|   stm32f427_437_429_439_tfbga216 IBIS Model
[IBIS ver]   4.2
[File name]  stm32f427_437_429_439_tfbga216.ibs
[File Rev]   1.3
[Date]   05-30-2014
[Source] Data Created at STMicroelectronics
[Notes]   File originated from ELDO simulations.
[Disclaimer]  This information is for modeling purpose only and is
   not guaranted. The information is subject to change without
   notice.
[Copyright] Copyright 2014 STMicroelectronics Inc.
[Component] stm32f427_437_429_439_tfbga216
[Manufacturer] STMicroelectronics
[Package]
| variable   typ   min   max
R_pkg   0.0   NA   NA
L_pkg   0.0H   NA   NA
C_pkg   0.0F   NA   NA
[Pin]   signal_name   model_name   R_pin   L_pin   C_pin
A3   PE2   io8p_arsudq_ft
A2   PE3   io8p_arsudq_ft
A1   PE4   io8p_arsudq_ft
B1   PE5   io8p_arsudq_ft
B2   PE6   io8p_arsudq_ft
G6   VSS   GND
F5   VDD   POWER
C1   VBAT   POWER
C2   PI8   io8p_arsudq_ft_v33
D1   PC13   io8p_arwsudq_ft_v33
E1   PC14   io8p_arwsudq_ft
F1   PC15   io8p_arsudq_ft
G5   VDD   POWER
E4   PI9   io8p_arsudq_ft
D5   PI10   io8p_arsudq_ft
F3   PI11   io8p_arsudq_ft
F2   VSS   GND
F4   VDD   POWER
D2   PF0   io8p_arsudq_i2cin_ft
E2   PF1   io8p_arsudq_i2cin_ft
G2   PF2   io8p_arsudq_ft
E3   PI12   io8p_arsudq_ft
G3   PI13   io8p_arsudq_ft
H3   PI14   io8p_arsudq_ft
H2   PF3   io8p_arwsudq_ft
J2   PF4   io8p_arwsudq_ft
K3   PF5   io8p_arwsudq_ft
H6   VSS   GND
H5   VDD   POWER
K2   PF6   io8p_arwsudq_ft
K1   PF7   io8p_arwsudq_ft
L3   PF8   io8p_arwsudq_ft
L2   PF9   io8p_arwsudq_ft
L1   PF10   io8p_arwsudq_ft
G1   PH0   io8p_arsudq_ft
H1   PH1   io8p_arsudq_ft
J1   NRST   ioreset_ft_v33
M2   PC0   io8p_ar3wsudq_ft
M3   PC1   io8p_ar3wsudq_ft
M4   PC2   io8p_ar3wsudq_ft
L4   PC3   io8p_ar3wsudq_ft
J5   VDD   POWER
J6   VSS   GND
M1   VSSA  GND
N1   VREFM   POWER
P1   VREFP   POWER
R1   VDDA   POWER
N3   PA0   io8p_ar3wsudq_ft_v33
N2   PA1   io8p_ar3wsudq_ft
P2   PA2   io8p_ar3wsudq_ft
K4   PH2   io8p_arsudq_ft
J4   PH3   io8p_arsudq_ft
H4   PH4   io8p_arsudq_i2cin_ft
J3   PH5   io8p_arsudq_i2cin_ft
R2   PA3   io8p_ar3wsudq_ft
K6   VSS   GND
L5   BYPASS_REG io8p_arsudq_ft_v33
K5   VDD   POWER
N4   PA4   io8p_ar3wsudq_ft
P4   PA5   io8p_ar3wsudq_ft
P3   PA6   io8p_ar3wsudq_ft
R3   PA7   io8p_ar3wsudq_ft
N5   PC4   io8p_ar3wsudq_ft
P5   PC5   io8p_ar3wsudq_ft
L7   VDD   POWER
L6   VSS   GND
R5   PB0   io8p_ar3wsudq_ft
R4   PB1   io8p_ar3wsudq_ft
M5   PB2   io8p_ar3wsudq_ft
G4   PI15   io8p_arsudq_ft
R6   PJ0   io8p_arsudq_ft
R7   PJ1   io8p_arsudq_ft
P7   PJ2   io8p_arsudq_ft
N8   PJ3   io8p_arsudq_ft
M9   PJ4   io8p_arsudq_ft
P8   PF11   io8p_arsudq_ft
M6   PF12   io8p_arsudq_ft
K7   VSS   GND
L8   VDD   POWER
N6   PF13   io8p_arsudq_ft
P6   PF14   io8p_arsudq_ft
M8   PF15   io8p_arsudq_ft
N7   PG0   io8p_arsudq_ft
M7   PG1   io8p_arsudq_ft
R8   PE7   io8p_arsudq_ft
N9   PE8   io8p_arsudq_ft
P9   PE9   io8p_arsudq_ft
K8   VSS   GND
L9   VDD   POWER
R9   PE10   io8p_arsudq_ft
P10   PE11   io8p_arsudq_ft
R10   PE12   io8p_arsudq_ft
R12   PE13   io8p_arsudq_ft
P11   PE14   io8p_arsudq_ft
R11   PE15   io8p_ar3wsudq_ft
P12   PB10   io8p_arsudq_i2cin_ft
R13   PB11   io8p_arsudq_i2cin_ft
L11   VCAP1   POWER
K9   VSS   GND
L10   VDD   POWER
M14   PJ5   io8p_arsudq_ft
P13   PH6   io8p_arsudq_ft
N13   PH7   io8p_arsudq_i2cin_ft
P14   PH8   io8p_arsudq_i2cin_ft
N14   PH9   io8p_arsudq_ft
p15   PH10   io8p_arsudq_ft
N15   PH11   io8p_arsudq_ft
M15   PH12   io8p_arsudq_ft
K10   VSS   GND
K11   VDD   POWER
L13   PB12   io8usb_id_otg_ft
K14   PB13   io8usb_vbus_otg_ft
R14   PB14   io8usb_lsfs_otg_ft
R15   PB15   io8usb_lsfs_otg_ft
L15   PD8   io8p_arsudq_ft
L14   PD9   io8p_arsudq_ft
K15   PD10   io8p_arsudq_ft
N10   PD11   io8p_arsudq_ft
M10   PD12   io8p_arsudq_ft
M11   PD13   io8p_arsudq_ft
J10   VSS   GND
J11   VDD   POWER
L12   PD14   io8p_arsudq_ft
K13   PD15   io8p_arsudq_ft
K12   PJ6   io8p_arsudq_ft
J12   PJ7   io8p_arsudq_ft
H12   PJ8   io8p_arsudq_ft
J13   PJ9   io8p_arsudq_ft
H13   PJ10   io8p_arsudq_ft
G12   PJ11   io8p_arsudq_ft
H11   VDD   POWER
H10   VSS   GND
G13   PK0   io8p_arsudq_ft
F12   PK1   io8p_arsudq_ft
F13   PK2   io8p_arsudq_ft
M13   PG2   io8p_arsudq_ft
M12   PG3   io8p_arsudq_ft
N12   PG4   io8p_arsudq_ft
N11   PG5   io8p_arsudq_ft
J15   PG6   io8p_arsudq_ft
J14   PG7   io8p_arsudq_ft
H14   PG8   io8p_arsudq_ft
G10   VSS   GND
G11   VDD   POWER
H15   PC6   io8p_arsudq_ft
G15   PC7   io8p_arsudq_ft
G14   PC8   io8p_arsudq_ft
F14   PC9   io8p_arsudq_i2cin_ft
F15   PA8   io8p_arsudq_i2cin_ft
E15   PA9   io8usb_vbus_otg_ft
D15   PA10   io8usb_id_otg_ft
C15   PA11   io8usb_lsfs_otg_ft
B15   PA12   io8usb_lsfs_otg_ft
A15   PA13   io8p_arsudq_ft
E11   VCAP2   POWER
F10   VSS   GND
F11   VDD   POWER
E12   PH13   io8p_arsudq_ft
E13   PH14   io8p_arsudq_ft
D13   PH15   io8p_arsudq_ft
E14   PI0   io8p_arsudq_ft
D14   PI1   io8p_arsudq_ft
C14   PI2   io8p_arsudq_ft
C13   PI3   io8p_arsudq_ft
F9   VSS   GND
E10   VDD   POWER
A14   PA14   io8p_arsudq_ft
A13   PA15   io8p_arsudq_ft
B14   PC10   io8p_arsudq_ft
B13   PC11   io8p_arsudq_ft
A12   PC12   io8p_arsudq_ft
B12   PD0   io8p_arsudq_ft
C12   PD1   io8p_arsudq_ft
D12   PD2   io8p_arsudq_ft
C11   PD3   io8p_arsudq_ft
D11   PD4   io8p_arsudq_ft
C10   PD5   io8p_arsudq_ft
F8   VSS   GND
E9   VDD   POWER
B11   PD6   io8p_arsudq_ft
A11   PD7   io8p_arsudq_ft
B10   PJ12   io8p_arsudq_ft
B9   PJ13   io8p_arsudq_ft
C9   PJ14   io8p_arsudq_ft
D10   PJ15   io8p_arsudq_ft
D9   PG9   io8p_arsudq_ft
C8   PG10   io8p_arsudq_ft
B8   PG11   io8p_arsudq_ft
C7   PG12   io8p_arsudq_ft
B3   PG13   io8p_arsudq_ft
A4   PG14   io8p_arsudq_ft
F7   VSS   GND
E8   VDD   POWER
D8   PK3   io8p_arsudq_ft
D7   PK4   io8p_arsudq_ft
C6   PK5   io8p_arsudq_ft
C5   PK6   io8p_arsudq_ft
C4   PK7   io8p_arsudq_ft
B7   PG15   io8p_arsudq_ft
A10   PB3   io8p_arsudq_ft
A9   PB4   io8p_arsudq_ft
A8   PB5   io8p_ar3wsudq_ft
B6   PB6   io8p_arsudq_i2cin_ft
B5   PB7   io8p_arsudq_i2cin_ft
E6   BOOT0   vpp_test_hv
A7   PB8   io8p_arsudq_i2cin_ft
B4   PB9   io8p_arsudq_i2cin_ft
A6   PE0   io8p_arsudq_ft
A5   PE1   io8p_arsudq_ft
F6   VSS   GND
E5   PDR_ON   io8p_arsudq_ft_v33
E7   VDD   POWER
C3   PI4   io8p_arsudq_ft
D3   PI5   io8p_arsudq_ft
D6   PI6   io8p_arsudq_ft
D4   PI7   io8p_arsudq_ft
[Diff Pin]   inv_pin   vdiff   tdelay_typ  tdelay_min  tdelay_max
R14   R15   200mV   NA   NA   NA
B15   C15   200mV   NA   NA   NA
[Model Selector] io8p_ar3wsudq_ft
io8p00_ar3wsudq_ft_pd_lv  "SPEED00 1P8V, PD=40kOhm"
io8p00_ar3wsudq_ft_pu_lv  "SPEED00 1P8V, PU=40kOhm"
io8p00_ar3wsudq_ft_lv   "SPEED00 1P8V"
io8p01_ar3wsudq_ft_pd_lv  "SPEED01 1P8V, PD=40kOhm"
io8p01_ar3wsudq_ft_pu_lv  "SPEED01 1P8V, PU=40kOhm"
io8p01_ar3wsudq_ft_lv  "SPEED01 1P8V"
io8p10_ar3wsudq_ft_pd_lv  "SPEED10 1P8V, PD=40kOhm"
io8p10_ar3wsudq_ft_pu_lv  "SPEED10 1P8V, PU=40kOhm"
io8p10_ar3wsudq_ft_lv  "SPEED10 1P8V"
io8p11_ar3wsudq_ft_pd_lv  "SPEED11 1P8V, PD=40kOhm"
io8p11_ar3wsudq_ft_pu_lv  "SPEED11 1P8V, PU=40kOhm"
io8p11_ar3wsudq_ft_lv  "SPEED11 1P8V"
io8p00_ar3wsudq_ft_pd  "SPEED00, PD=40kOhm"
io8p00_ar3wsudq_ft_pu  "SPEED00, PU=40kOhm"
io8p00_ar3wsudq_ft  "SPEED00"
io8p01_ar3wsudq_ft_pd  "SPEED01, PD=40kOhm"
io8p01_ar3wsudq_ft_pu  "SPEED01, PU=40kOhm"
io8p01_ar3wsudq_ft  "SPEED01"
io8p10_ar3wsudq_ft_pd  "SPEED10, PD=40kOhm"
io8p10_ar3wsudq_ft_pu  "SPEED10, PU=40kOhm"
io8p10_ar3wsudq_ft  "SPEED10"
io8p11_ar3wsudq_ft_pd  "SPEED11, PD=40kOhm"
io8p11_ar3wsudq_ft_pu  "SPEED11, PU=40kOhm"
io8p11_ar3wsudq_ft  "SPEED11"
[Model Selector] io8p_ar3wsudq_ft_v33
io8p00_ar3wsudq_ft_v33_pd_lv  "SPEED00 1P8V, PD=40kOhm"
io8p00_ar3wsudq_ft_v33_pu_lv  "SPEED00 1P8V, PU=40kOhm"
io8p00_ar3wsudq_ft_v33_lv  "SPEED00 1P8V"
io8p01_ar3wsudq_ft_v33_pd_lv  "SPEED01 1P8V, PD=40kOhm"
io8p01_ar3wsudq_ft_v33_pu_lv  "SPEED01 1P8V, PU=40kOhm"
io8p01_ar3wsudq_ft_v33_lv  "SPEED01 1P8V"
io8p10_ar3wsudq_ft_v33_pd_lv  "SPEED10 1P8V, PD=40kOhm"
io8p10_ar3wsudq_ft_v33_pu_lv  "SPEED10 1P8V, PU=40kOhm"
io8p10_ar3wsudq_ft_v33_lv  "SPEED10 1P8V"
io8p11_ar3wsudq_ft_v33_pd_lv  "SPEED11 1P8V, PD=40kOhm"
io8p11_ar3wsudq_ft_v33_pu_lv  "SPEED11 1P8V, PU=40kOhm"
io8p11_ar3wsudq_ft_v33_lv  "SPEED11 1P8V"
io8p00_ar3wsudq_ft_v33_pd  "SPEED00, PD=40kOhm"
io8p00_ar3wsudq_ft_v33_pu  "SPEED00, PU=40kOhm"
io8p00_ar3wsudq_ft_v33  "SPEED00"
io8p01_ar3wsudq_ft_v33_pd  "SPEED01, PD=40kOhm"
io8p01_ar3wsudq_ft_v33_pu  "SPEED01, PU=40kOhm"
io8p01_ar3wsudq_ft_v33  "SPEED01"
io8p10_ar3wsudq_ft_v33_pd  "SPEED10, PD=40kOhm"
io8p10_ar3wsudq_ft_v33_pu  "SPEED10, PU=40kOhm"
io8p10_ar3wsudq_ft_v33  "SPEED10"
io8p11_ar3wsudq_ft_v33_pd  "SPEED11, PD=40kOhm"
io8p11_ar3wsudq_ft_v33_pu  "SPEED11, PU=40kOhm"
io8p11_ar3wsudq_ft_v33  "SPEED11"
[Model Selector] io8p_arsudq_ft
io8p00_arsudq_ft_pd_lv  "SPEED00 1P8V, PD=40kOhm"
io8p00_arsudq_ft_pu_lv  "SPEED00 1P8V, PU=40kOhm"
io8p00_arsudq_ft_lv  "SPEED00 1P8V"
io8p01_arsudq_ft_pd_lv  "SPEED01 1P8V, PD=40kOhm"
io8p01_arsudq_ft_pu_lv  "SPEED01 1P8V, PU=40kOhm"
io8p01_arsudq_ft_lv  "SPEED01 1P8V"
io8p10_arsudq_ft_pd_lv  "SPEED10 1P8V, PD=40kOhm"
io8p10_arsudq_ft_pu_lv  "SPEED10 1P8V, PU=40kOhm"
io8p10_arsudq_ft_lv  "SPEED10 1P8V"
io8p11_arsudq_ft_pd_lv  "SPEED11 1P8V, PD=40kOhm"
io8p11_arsudq_ft_pu_lv  "SPEED11 1P8V, PU=40kOhm"
io8p11_arsudq_ft_lv  "SPEED11 1P8V"
io8p00_arsudq_ft_pd  "SPEED00, PD=40kOhm"
io8p00_arsudq_ft_pu  "SPEED00, PU=40kOhm"
io8p00_arsudq_ft  "SPEED00"
io8p01_arsudq_ft_pd  "SPEED01, PD=40kOhm"
io8p01_arsudq_ft_pu  "SPEED01, PU=40kOhm"
io8p01_arsudq_ft  "SPEED01"
io8p10_arsudq_ft_pd  "SPEED10, PD=40kOhm"
io8p10_arsudq_ft_pu  "SPEED10, PU=40kOhm"
io8p10_arsudq_ft  "SPEED10"
io8p11_arsudq_ft_pd  "SPEED11, PD=40kOhm"
io8p11_arsudq_ft_pu  "SPEED11, PU=40kOhm"
io8p11_arsudq_ft  "SPEED11"
[Model Selector] io8p_arsudq_ft_v33
io8p00_arsudq_ft_v33_pd_lv  "SPEED00 1P8V, PD=40kOhm"
io8p00_arsudq_ft_v33_pu_lv  "SPEED00 1P8V, PU=40kOhm"
io8p00_arsudq_ft_v33_lv  "SPEED00 1P8V"
io8p01_arsudq_ft_v33_pd_lv  "SPEED01 1P8V, PD=40kOhm"
io8p01_arsudq_ft_v33_pu_lv  "SPEED01 1P8V, PU=40kOhm"
io8p01_arsudq_ft_v33_lv  "SPEED01 1P8V"
io8p10_arsudq_ft_v33_pd_lv  "SPEED10 1P8V, PD=40kOhm"
io8p10_arsudq_ft_v33_pu_lv  "SPEED10 1P8V, PU=40kOhm"
io8p10_arsudq_ft_v33_lv  "SPEED10 1P8V"
io8p11_arsudq_ft_v33_pd_lv  "SPEED11 1P8V, PD=40kOhm"
io8p11_arsudq_ft_v33_pu_lv  "SPEED11 1P8V, PU=40kOhm"
io8p11_arsudq_ft_v33_lv  "SPEED11 1P8V"
io8p00_arsudq_ft_v33_pd  "SPEED00, PD=40kOhm"
io8p00_arsudq_ft_v33_pu  "SPEED00, PU=40kOhm"
io8p00_arsudq_ft_v33  "SPEED00"
io8p01_arsudq_ft_v33_pd  "SPEED01, PD=40kOhm"
io8p01_arsudq_ft_v33_pu  "SPEED01, PU=40kOhm"
io8p01_arsudq_ft_v33  "SPEED01"
io8p10_arsudq_ft_v33_pd  "SPEED10, PD=40kOhm"
io8p10_arsudq_ft_v33_pu  "SPEED10, PU=40kOhm"
io8p10_arsudq_ft_v33  "SPEED10"
io8p11_arsudq_ft_v33_pd  "SPEED11, PD=40kOhm"
io8p11_arsudq_ft_v33_pu  "SPEED11, PU=40kOhm"
io8p11_arsudq_ft_v33  "SPEED11"
[Model Selector] io8p_arsudq_i2cin_ft
io8p00_arsudq_i2cin_ft_pd_lv  "SPEED00 1P8V, PD=40kOhm"
io8p00_arsudq_i2cin_ft_pu_lv  "SPEED00 1P8V, PU=40kOhm"
io8p00_arsudq_i2cin_ft_lv  "SPEED00 1P8V"
io8p01_arsudq_i2cin_ft_pd_lv  "SPEED01 1P8V, PD=40kOhm"
io8p01_arsudq_i2cin_ft_pu_lv  "SPEED01 1P8V, PU=40kOhm"
io8p01_arsudq_i2cin_ft_lv  "SPEED01 1P8V"
io8p10_arsudq_i2cin_ft_pd_lv  "SPEED10 1P8V, PD=40kOhm"
io8p10_arsudq_i2cin_ft_pu_lv  "SPEED10 1P8V, PU=40kOhm"
io8p10_arsudq_i2cin_ft_lv  "SPEED10 1P8V"
io8p11_arsudq_i2cin_ft_pd_lv  "SPEED11 1P8V, PD=40kOhm"
io8p11_arsudq_i2cin_ft_pu_lv  "SPEED11 1P8V, PU=40kOhm"
io8p11_arsudq_i2cin_ft_lv  "SPEED11 1P8V"
io8p00_arsudq_i2cin_ft_pd  "SPEED00, PD=40kOhm"
io8p00_arsudq_i2cin_ft_pu  "SPEED00, PU=40kOhm"
io8p00_arsudq_i2cin_ft  "SPEED00"
io8p01_arsudq_i2cin_ft_pd  "SPEED01, PD=40kOhm"
io8p01_arsudq_i2cin_ft_pu  "SPEED01, PU=40kOhm"
io8p01_arsudq_i2cin_ft  "SPEED01"
io8p10_arsudq_i2cin_ft_pd  "SPEED10, PD=40kOhm"
io8p10_arsudq_i2cin_ft_pu  "SPEED10, PU=40kOhm"
io8p10_arsudq_i2cin_ft  "SPEED10"
io8p11_arsudq_i2cin_ft_pd  "SPEED11, PD=40kOhm"
io8p11_arsudq_i2cin_ft_pu  "SPEED11, PU=40kOhm"
io8p11_arsudq_i2cin_ft  "SPEED11"
[Model Selector] io8p_arwsudq_ft
io8p00_arwsudq_ft_pd_lv  "SPEED00 1P8V, PD=40kOhm"
io8p00_arwsudq_ft_pu_lv  "SPEED00 1P8V, PU=40kOhm"
io8p00_arwsudq_ft_lv  "SPEED00 1P8V"
io8p01_arwsudq_ft_pd_lv  "SPEED01 1P8V, PD=40kOhm"
io8p01_arwsudq_ft_pu_lv  "SPEED01 1P8V, PU=40kOhm"
io8p01_arwsudq_ft_lv  "SPEED01 1P8V"
io8p10_arwsudq_ft_pd_lv  "SPEED10 1P8V, PD=40kOhm"
io8p10_arwsudq_ft_pu_lv  "SPEED10 1P8V, PU=40kOhm"
io8p10_arwsudq_ft_lv  "SPEED10 1P8V"
io8p11_arwsudq_ft_pd_lv  "SPEED11 1P8V, PD=40kOhm"
io8p11_arwsudq_ft_pu_lv  "SPEED11 1P8V, PU=40kOhm"
io8p11_arwsudq_ft_lv  "SPEED11 1P8V"
io8p00_arwsudq_ft_pd  "SPEED00, PD=40kOhm"
io8p00_arwsudq_ft_pu  "SPEED00, PU=40kOhm"
io8p00_arwsudq_ft  "SPEED00"
io8p01_arwsudq_ft_pd  "SPEED01, PD=40kOhm"
io8p01_arwsudq_ft_pu  "SPEED01, PU=40kOhm"
io8p01_arwsudq_ft  "SPEED01"
io8p10_arwsudq_ft_pd  "SPEED10, PD=40kOhm"
io8p10_arwsudq_ft_pu  "SPEED10, PU=40kOhm"
io8p10_arwsudq_ft  "SPEED10"
io8p11_arwsudq_ft_pd  "SPEED11, PD=40kOhm"
io8p11_arwsudq_ft_pu  "SPEED11, PU=40kOhm"
io8p11_arwsudq_ft  "SPEED11"
[Model Selector] io8p_arwsudq_ft_v33
io8p00_arwsudq_ft_v33_pd_lv  "SPEED00 1P8V, PD=40kOhm"
io8p00_arwsudq_ft_v33_pu_lv  "SPEED00 1P8V, PU=40kOhm"
io8p00_arwsudq_ft_v33_lv  "SPEED00 1P8V"
io8p01_arwsudq_ft_v33_pd_lv  "SPEED01 1P8V, PD=40kOhm"
io8p01_arwsudq_ft_v33_pu_lv  "SPEED01 1P8V, PU=40kOhm"
io8p01_arwsudq_ft_v33_lv  "SPEED01 1P8V"
io8p10_arwsudq_ft_v33_pd_lv  "SPEED10 1P8V, PD=40kOhm"
io8p10_arwsudq_ft_v33_pu_lv  "SPEED10 1P8V, PU=40kOhm"
io8p10_arwsudq_ft_v33_lv  "SPEED10 1P8V"
io8p11_arwsudq_ft_v33_pd_lv  "SPEED11 1P8V, PD=40kOhm"
io8p11_arwsudq_ft_v33_pu_lv  "SPEED11 1P8V, PU=40kOhm"
io8p11_arwsudq_ft_v33_lv  "SPEED11 1P8V"
io8p00_arwsudq_ft_v33_pd  "SPEED00, PD=40kOhm"
io8p00_arwsudq_ft_v33_pu  "SPEED00, PU=40kOhm"
io8p00_arwsudq_ft_v33  "SPEED00"
io8p01_arwsudq_ft_v33_pd  "SPEED01, PD=40kOhm"
io8p01_arwsudq_ft_v33_pu  "SPEED01, PU=40kOhm"
io8p01_arwsudq_ft_v33  "SPEED01"
io8p10_arwsudq_ft_v33_pd  "SPEED10, PD=40kOhm"
io8p10_arwsudq_ft_v33_pu  "SPEED10, PU=40kOhm"
io8p10_arwsudq_ft_v33  "SPEED10"
io8p11_arwsudq_ft_v33_pd  "SPEED11, PD=40kOhm"
io8p11_arwsudq_ft_v33_pu  "SPEED11, PU=40kOhm"
io8p11_arwsudq_ft_v33  "SPEED11"
[Model Selector] io8usb_id_otg_ft
io8p00_id_otg_ft_pd_lv  "SPEED00 1P8V, PD=14kOhm"
io8p00_id_otg_ft_pu_lv  "SPEED00 1P8V, PU=14kOhm"
io8p00_id_otg_ft_lv  "SPEED00 1P8V"
io8p01_id_otg_ft_pd_lv  "SPEED01 1P8V, PD=14kOhm"
io8p01_id_otg_ft_pu_lv  "SPEED01 1P8V, PU=14kOhm"
io8p01_id_otg_ft_lv  "SPEED01 1P8V"
io8p10_id_otg_ft_pd_lv  "SPEED10 1P8V, PD=14kOhm"
io8p10_id_otg_ft_pu_lv  "SPEED10 1P8V, PU=14kOhm"
io8p10_id_otg_ft_lv  "SPEED10 1P8V"
io8p11_id_otg_ft_pd_lv  "SPEED11 1P8V, PD=14kOhm"
io8p11_id_otg_ft_pu_lv  "SPEED11 1P8V, PU=14kOhm"
io8p11_id_otg_ft_lv  "SPEED11 1P8V"
io8p00_id_otg_ft_pd  "SPEED00, PD=14kOhm"
io8p00_id_otg_ft_pu  "SPEED00, PU=14kOhm"
io8p00_id_otg_ft  "SPEED00"
io8p01_id_otg_ft_pd  "SPEED01, PD=14kOhm"
io8p01_id_otg_ft_pu  "SPEED01, PU=14kOhm"
io8p01_id_otg_ft  "SPEED01"
io8p10_id_otg_ft_pd  "SPEED10, PD=14kOhm"
io8p10_id_otg_ft_pu  "SPEED10, PU=14kOhm"
io8p10_id_otg_ft  "SPEED10"
io8p11_id_otg_ft_pd  "SPEED11, PD=14kOhm"
io8p11_id_otg_ft_pu  "SPEED11, PU=14kOhm"
io8p11_id_otg_ft  "SPEED11"
[Model Selector] io8usb_lsfs_otg_ft
io8usb_ls_otg_ft_dpdn_pd  "LS USB DP/DN IO + PD=20kOhm"
io8usb_ls_otg_ft_dpdn_pupu2  "LS USB DP/DN IO + PU/PU2=2.2kOhm"
io8usb_ls_otg_ft_dpdn_pu2  "LS USB DP/DN IO + PU2=1.2kOhm"
io8usb_ls_otg_ft_dpdn_pu  "LS USB DP/DN IO + PU=1.2kOhm"
io8usb_ls_otg_ft_dpdn  "LS USB DP/DN IO"
io8usb_fs_otg_ft_dpdn_pd  "HS USB DP/DN IO + PD=20kOhm"
io8usb_fs_otg_ft_dpdn_pupu2  "HS USB DP/DN IO + PU/PU2=2.2kOhm"
io8usb_fs_otg_ft_dpdn_pu2  "HS USB DP/DN IO + PU2=1.2kOhm"
io8usb_fs_otg_ft_dpdn_pu  "HS USB DP/DN IO + PU=1.2kOhm"
io8usb_fs_otg_ft_dpdn  "HS USB DP/DN IO"
io8p00_lsfs_otg_ft_pd_lv  "SPEED00 1P8V, PD=40kOhm"
io8p00_lsfs_otg_ft_pu_lv  "SPEED00 1P8V, PU=40kOhm"
io8p00_lsfs_otg_ft_lv  "SPEED00 1P8V"
io8p01_lsfs_otg_ft_pd_lv  "SPEED01 1P8V, PD=40kOhm"
io8p01_lsfs_otg_ft_pu_lv  "SPEED01 1P8V, PU=40kOhm"
io8p01_lsfs_otg_ft_lv  "SPEED01 1P8V"
io8p10_lsfs_otg_ft_pd_lv  "SPEED10 1P8V, PD=40kOhm"
io8p10_lsfs_otg_ft_pu_lv  "SPEED10 1P8V, PU=40kOhm"
io8p10_lsfs_otg_ft_lv  "SPEED10 1P8V"
io8p11_lsfs_otg_ft_pd_lv  "SPEED11 1P8V, PD=40kOhm"
io8p11_lsfs_otg_ft_pu_lv  "SPEED11 1P8V, PU=40kOhm"
io8p11_lsfs_otg_ft_lv  "SPEED11 1P8V"
io8p00_lsfs_otg_ft_pd  "SPEED00, PD=40kOhm"
io8p00_lsfs_otg_ft_pu  "SPEED00, PU=40kOhm"
io8p00_lsfs_otg_ft  "SPEED00"
io8p01_lsfs_otg_ft_pd  "SPEED01, PD=40kOhm"
io8p01_lsfs_otg_ft_pu  "SPEED01, PU=40kOhm"
io8p01_lsfs_otg_ft  "SPEED01"
io8p10_lsfs_otg_ft_pd  "SPEED10, PD=40kOhm"
io8p10_lsfs_otg_ft_pu  "SPEED10, PU=40kOhm"
io8p10_lsfs_otg_ft  "SPEED10"
io8p11_lsfs_otg_ft_pd  "SPEED11, PD=40kOhm"
io8p11_lsfs_otg_ft_pu  "SPEED11, PU=40kOhm"
io8p11_lsfs_otg_ft  "SPEED11"
[Model Selector] io8usb_vbus_otg_ft
io8psenb_vbus_otg_ft  "VBUS PULSE, SENSE VB"
io8psenab_vbus_otg_ft  "VBUS PULSE, SENSE VA and VB"
io8psena_vbus_otg_ft  "VBUS PULSE, SENSE VA"
io8psen_vbus_otg_ft  "VBUS PULSE"
io8p00_vbus_otg_ft_pd_lv  "SPEED00 1P8V, PD=40kOhm"
io8p00_vbus_otg_ft_pu_lv  "SPEED00 1P8V, PU=40kOhm"
io8p00_vbus_otg_ft_lv  "SPEED00 1P8V"
io8p01_vbus_otg_ft_pd_lv  "SPEED01 1P8V, PD=40kOhm"
io8p01_vbus_otg_ft_pu_lv  "SPEED01 1P8V, PU=40kOhm"
io8p01_vbus_otg_ft_lv  "SPEED01 1P8V"
io8p10_vbus_otg_ft_pd_lv  "SPEED10 1P8V, PD=40kOhm"
io8p10_vbus_otg_ft_pu_lv  "SPEED10 1P8V, PU=40kOhm"
io8p10_vbus_otg_ft_lv  "SPEED10 1P8V"
io8p11_vbus_otg_ft_pd_lv  "SPEED11 1P8V, PD=40kOhm"
io8p11_vbus_otg_ft_pu_lv  "SPEED11 1P8V, PU=40kOhm"
io8p11_vbus_otg_ft_lv  "SPEED11 1P8V"
io8p00_vbus_otg_ft_pd  "SPEED00, PD=40kOhm"
io8p00_vbus_otg_ft_pu  "SPEED00, PU=40kOhm"
io8p00_vbus_otg_ft  "SPEED00"
io8p01_vbus_otg_ft_pd  "SPEED01, PD=40kOhm"
io8p01_vbus_otg_ft_pu  "SPEED01, PU=40kOhm"
io8p01_vbus_otg_ft  "SPEED01"
io8p10_vbus_otg_ft_pd  "SPEED10, PD=40kOhm"
io8p10_vbus_otg_ft_pu  "SPEED10, PU=40kOhm"
io8p10_vbus_otg_ft  "SPEED10"
io8p11_vbus_otg_ft_pd  "SPEED11, PD=40kOhm"
io8p11_vbus_otg_ft_pu  "SPEED11, PU=40kOhm"
io8p11_vbus_otg_ft  "SPEED11"
[Model Selector] ioreset_ft_v33
ioreset_ft_v33_pu_lv  "ioreset 1P8V + PU=40kOhm"
ioreset_ft_v33_nopu_lv  "ioreset 1P8V"
ioreset_ft_v33_pu  "ioreset + PU=40kOhm"
ioreset_ft_v33_nopu  "ioreset"
[Model Selector] vpp_test_hv
vpp_test_hv_2p4  "Input Buffer 1P8V"
vpp_test_hv_3p3  "Input Buffer"
| Models and submodels in the file (260): io8p00_ar3wsudq_ft_pd_lv (I/O), io8p00_ar3wsudq_ft_pu_lv (I/O), io8p00_ar3wsudq_ft_lv (I/O), io8p01_ar3wsudq_ft_pd_lv (I/O), io8p01_ar3wsudq_ft_pu_lv (I/O), io8p01_ar3wsudq_ft_lv (I/O), io8p10_ar3wsudq_ft_pd_lv (I/O), io8p10_ar3wsudq_ft_pu_lv (I/O), io8p10_ar3wsudq_ft_lv (I/O), io8p11_ar3wsudq_ft_pd_lv (I/O), io8p11_ar3wsudq_ft_pu_lv (I/O), io8p11_ar3wsudq_ft_lv (I/O), io8p00_ar3wsudq_ft_pd (I/O), io8p00_ar3wsudq_ft_pu (I/O), io8p00_ar3wsudq_ft (I/O), io8p01_ar3wsudq_ft_pd (I/O), io8p01_ar3wsudq_ft_pu (I/O), io8p01_ar3wsudq_ft (I/O), io8p10_ar3wsudq_ft_pd (I/O), io8p10_ar3wsudq_ft_pu (I/O), io8p10_ar3wsudq_ft (I/O), io8p11_ar3wsudq_ft_pd (I/O), io8p11_ar3wsudq_ft_pu (I/O), io8p11_ar3wsudq_ft (I/O), io8p00_ar3wsudq_ft_v33_pd_lv (I/O), io8p00_ar3wsudq_ft_v33_pu_lv (I/O), io8p00_ar3wsudq_ft_v33_lv (I/O), io8p01_ar3wsudq_ft_v33_pd_lv (I/O), io8p01_ar3wsudq_ft_v33_pu_lv (I/O), io8p01_ar3wsudq_ft_v33_lv (I/O), io8p10_ar3wsudq_ft_v33_pd_lv (I/O), io8p10_ar3wsudq_ft_v33_pu_lv (I/O), io8p10_ar3wsudq_ft_v33_lv (I/O), io8p11_ar3wsudq_ft_v33_pd_lv (I/O), io8p11_ar3wsudq_ft_v33_pu_lv (I/O), io8p11_ar3wsudq_ft_v33_lv (I/O), io8p00_ar3wsudq_ft_v33_pd (I/O), io8p00_ar3wsudq_ft_v33_pu (I/O), io8p00_ar3wsudq_ft_v33 (I/O), io8p01_ar3wsudq_ft_v33_pd (I/O), io8p01_ar3wsudq_ft_v33_pu (I/O), io8p01_ar3wsudq_ft_v33 (I/O), io8p10_ar3wsudq_ft_v33_pd (I/O), io8p10_ar3wsudq_ft_v33_pu (I/O), io8p10_ar3wsudq_ft_v33 (I/O), io8p11_ar3wsudq_ft_v33_pd (I/O), io8p11_ar3wsudq_ft_v33_pu (I/O), io8p11_ar3wsudq_ft_v33 (I/O), io8p00_arsudq_ft_pd_lv (I/O), io8p00_arsudq_ft_pu_lv (I/O), io8p00_arsudq_ft_lv (I/O), io8p01_arsudq_ft_pd_lv (I/O), io8p01_arsudq_ft_pu_lv (I/O), io8p01_arsudq_ft_lv (I/O), io8p10_arsudq_ft_pd_lv (I/O), io8p10_arsudq_ft_pu_lv (I/O), io8p10_arsudq_ft_lv (I/O), io8p11_arsudq_ft_pd_lv (I/O), io8p11_arsudq_ft_pu_lv (I/O), io8p11_arsudq_ft_lv (I/O), io8p00_arsudq_ft_pd (I/O), io8p00_arsudq_ft_pu (I/O), io8p00_arsudq_ft (I/O), io8p01_arsudq_ft_pd (I/O), io8p01_arsudq_ft_pu (I/O), io8p01_arsudq_ft (I/O), io8p10_arsudq_ft_pd (I/O), io8p10_arsudq_ft_pu (I/O), io8p10_arsudq_ft (I/O), io8p11_arsudq_ft_pd (I/O), io8p11_arsudq_ft_pu (I/O), io8p11_arsudq_ft (I/O), io8p00_arsudq_ft_v33_pd_lv (I/O), io8p00_arsudq_ft_v33_pu_lv (I/O), io8p00_arsudq_ft_v33_lv (I/O), io8p01_arsudq_ft_v33_pd_lv (I/O), io8p01_arsudq_ft_v33_pu_lv (I/O), io8p01_arsudq_ft_v33_lv (I/O), io8p10_arsudq_ft_v33_pd_lv (I/O), io8p10_arsudq_ft_v33_pu_lv (I/O)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
